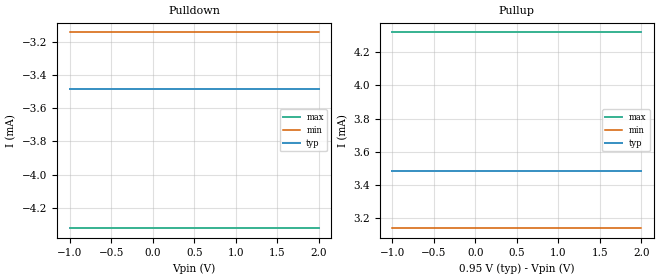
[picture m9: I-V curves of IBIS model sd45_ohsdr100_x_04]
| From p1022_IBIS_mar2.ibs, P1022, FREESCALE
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[Model]   sd45_ohsdr100_x_04
Model_type 3-state
Enable Active-High
Polarity Non-Inverting
|   TYP   MIN   MAX
C_comp   0.00pF   0.00pF   0.00pF
[Model Spec]
Vmeas   0.475   0.425   0.605
[Temperature Range] 65   125   -40
[Voltage Range]   0.95   0.85   1.21
[Pullup]
|   Vout(V)   TYP   WCS   BCS
-1V       3.486mA    3.14mA     4.319mA
2V        3.486mA    3.14mA     4.319mA
[Pulldown]
|   Vout(V)   TYP   WCS   BCS
-1V       -3.486mA   -3.142mA   -4.323mA
2V        -3.486mA   -3.142mA   -4.323mA
[GND Clamp]
|   Vout(V)   TYP   WCS   BCS
-1V       0A         0A         0A
1V        0A         0A         0A
[POWER Clamp]
|   Vout(V)   TYP   WCS   BCS
-1V       0A         0A         0A
0V        0A         0A         0A
[Ramp]
R_load=50
dV/dt_r  2.9887e-01/6.4040e-11  2.6861e-01/6.5155e-11  3.8214e-01/6.5744e-11
dV/dt_f  2.9887e-01/6.6355e-11  2.6861e-01/6.7761e-11  3.8218e-01/6.7348e-11
|[End   sd45_ohsdr100_x_04
